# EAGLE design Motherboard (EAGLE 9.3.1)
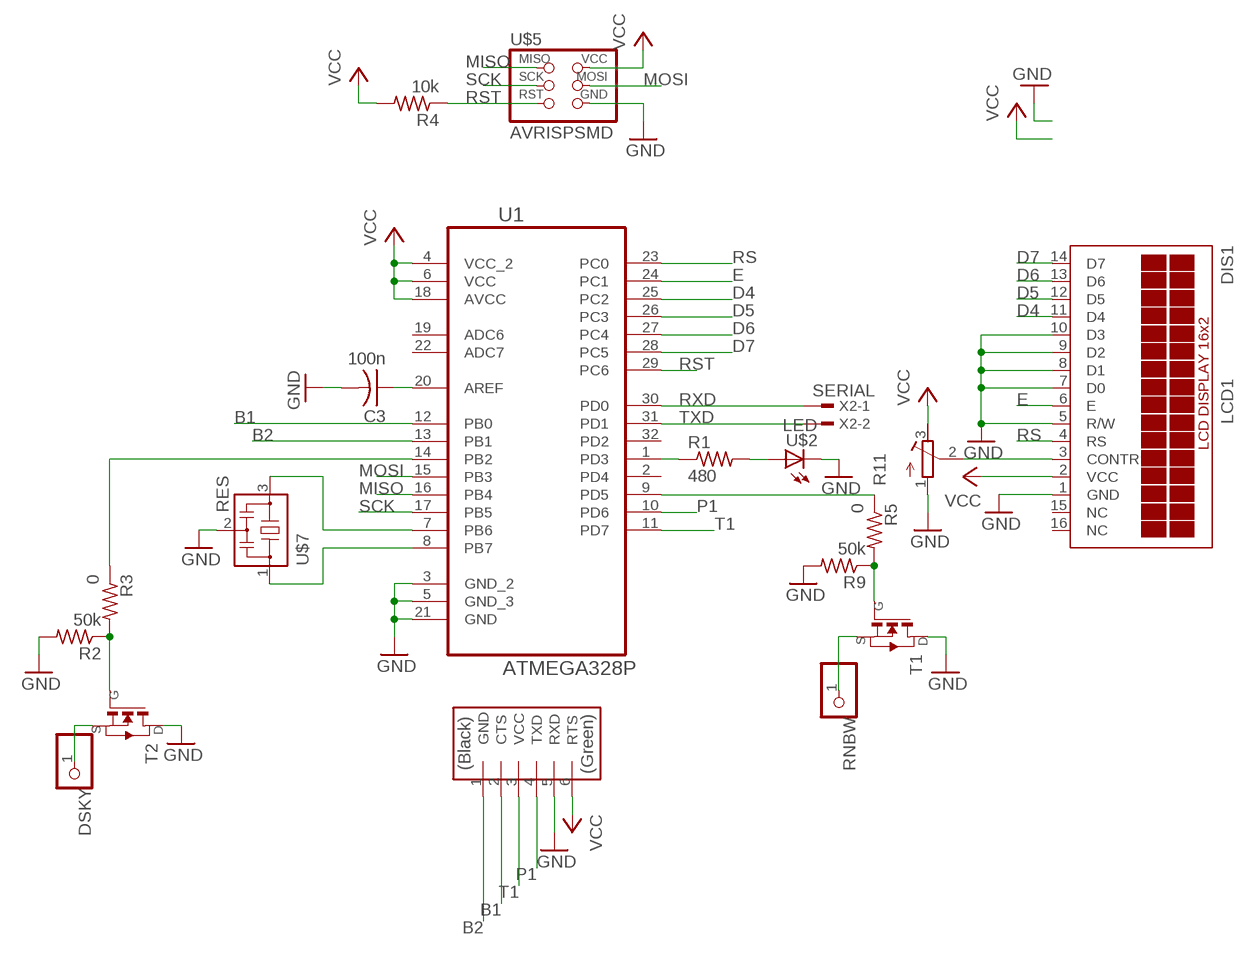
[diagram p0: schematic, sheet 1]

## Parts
C3  100n  CAP-US1206FAB  [C1206FAB]
DIS1  LCD1  TUXGR_16X2_R2  [TUXGR_16X2_R2]
DSKY  PINHD-1X1  [1X01]
R1  480  RES-US1206FAB  [R1206FAB]
R2  50k  RES-US1206FAB  [R1206FAB]
R3  0  RES-US1206FAB  [R1206FAB]
R4  10k  RES-US1206FAB  [R1206FAB]
R5  0  RES-US1206FAB  [R1206FAB]
R9  50k  RES-US1206FAB  [R1206FAB]
R11  R-TRIMM4G/J  [RTRIM4G/J]
RNBW  PINHD-1X1  [1X01]
T1  NMOSFETSOT23  [SOT-23]
T2  NMOSFETSOT23  [SOT-23]
U1  ATMEGA328P  ATMEGA328P-AU  [QFP80P900X900X120-32N]
U$1  FTDI-SMD-HEADER  [1X06SMD]
U$2  LED  LEDFAB1206  [LED1206FAB]
U$5  AVRISPSMD  [2X03SMD]
U$7  RES  RESONATOR  [EFOBM]
X2  SERIAL  TSW-101-07-G-D  [TSW-101-XX-G-D]

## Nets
B1: U1.12(PB0) U$1.2(CTS)
B2: U1.13(PB1) U$1.1(GND)
D4: DIS1.11(D4) U1.25(PC2)
D5: DIS1.12(D5) U1.26(PC3)
D6: DIS1.13(D6) U1.27(PC4)
D7: DIS1.14(D7) U1.28(PC5)
E: DIS1.6(E) U1.24(PC1)
GND: C3.2 DIS1.1(GND) DIS1.5(R/W) DIS1.7(D0) DIS1.8(D1) DIS1.9(D2) DIS1.10(D3) R2.2 R9.2 R11.1(A) T1.1(D) T2.1(D) U1.3(GND_2) U1.5(GND_3) U1.21(GND) U$1.5(RXD) U$2.2(C) U$5.6(GND) U$7.2
MISO: U1.16(PB4) U$5.1(MISO)
MOSI: U1.15(PB3) U$5.4(MOSI)
N$1: DIS1.3(CONTR) R11.2(S)
N$2: U1.7(PB6) U$7.3
N$3: C3.1 U1.20(AREF)
N$4: R1.1 U1.1(PD3)
N$6: R3.1 U1.14(PB2)
N$7: R1.2 U$2.1(A)
N$9: R5.1 U1.9(PD5)
N$11: R2.1 R3.2 T2.3(G)
N$12: R5.2 R9.1 T1.3(G)
N$19: RNBW.1 T1.2(S)
N$21: U1.8(PB7) U$7.1
N$22: DSKY.1 T2.2(S)
P1: U1.10(PD6) U$1.4(TXD)
RS: DIS1.4(RS) U1.23(PC0)
RST: R4.1 U1.29(PC6) U$5.5(RST)
RXD: U1.30(PD0) X2.1
SCK: U1.17(PB5) U$5.3(SCK)
T1: U1.11(PD7) U$1.3(VCC)
TXD: U1.31(PD1) X2.2
VCC: DIS1.2(VCC) R4.2 R11.3(E) U1.4(VCC_2) U1.6(VCC) U1.18(AVCC) U$1.6(RTS) U$5.2(VCC)
Unconnected: DIS1.15(NC) DIS1.16(NC) U1.2(PD4) U1.19(ADC6) U1.22(ADC7) U1.32(PD2)

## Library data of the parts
C3 = fab:CAP-US
DIS1 = lcd16:TUXGR_16X2_R2: Tuxgraphics LCD display 16x2 characters reflective, without background light Source: tuxgr_12x2_r2.pdf; OC_FARNELL: unknown; OC_NEWARK: unknown
DSKY RNBW = pinhead:PINHD-1X1: PIN HEADER
R1-R5 R9 = fab:RES-US: Resistor (US Symbol)
R11 = rcl:R-TRIMM: Trimm resistor; SPICEMODEL: X; SPICEPREFIXL: POT
T1 T2 = fab:NMOSFET: MOS FET
U1 = Atmel_By_element14_Batch_1-00:ATMEGA328P-AU: 8-bit Microcontroller with In-System Programmable Flash; MPN: ATMEGA328P-AU; OC_FARNELL: 1715486; OC_NEWARK: 14R4631; PACKAGE: TQFP-32; SUPPLIER: Atmel
U$1 = fab:FTDI-SMD-HEADER
U$2 = fab:LED: LED
U$5 = fab:AVRISP
U$7 = fab:RESONATOR
X2 = con-samtec:TSW-101-*-G: THROUGH-HOLE .025" SQ POST HEADER; MF: Samtec Inc.; MPN: TSW-101-07-G-D

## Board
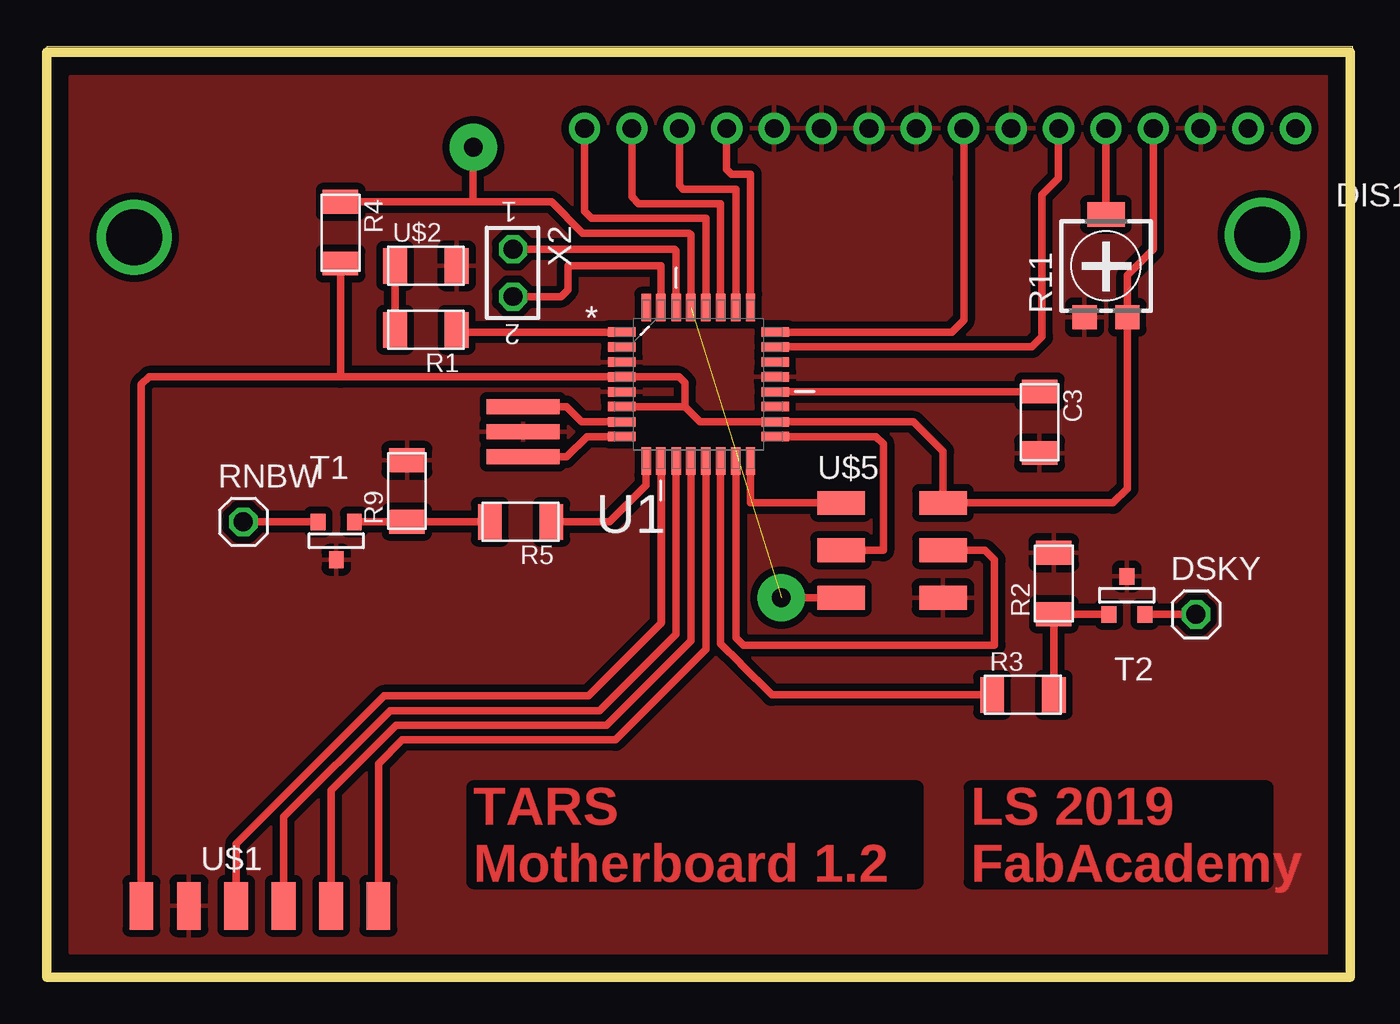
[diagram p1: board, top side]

Size 70 x 49.84 mm. Coordinates in mm from the lower left corner, seen from the top.
Outline: 0,0 70,0 70,49.84 0,49.84 0,0
Copper layers (1*16): Top 0.035mm / dielectric 1.5mm / Bottom 0.035mm
Design rules "default *": minimum track width 16mil, minimum drill 0.35mm, track to track 15mil, track to pad 15mil, pad to pad 15mil, via to via 15mil, smd to smd 15mil, copper to edge 40mil, drill to drill 6mil, minimum pad ring 10mil, minimum via ring 8mil, stop-mask expansion 4mil, vias tented up to drill 0mil, thermal gap 16mil
Milling: 4 lines

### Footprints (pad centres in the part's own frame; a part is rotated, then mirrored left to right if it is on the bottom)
C1206FAB = smd 1.27 x 1.905: 1 -1.651,0; 2 1.651,0
TUXGR_16X2_R2 = drill 1 pad 1.676: 1 -26.92,15.5; 2 -24.38,15.5; 3 -21.84,15.5; 4 -19.3,15.5; 5 -16.76,15.5; 6 -14.22,15.5; 7 -11.68,15.5; 8 -9.14,15.5; 9 -6.6,15.5; 10 -4.06,15.5; 11 -1.52,15.5; 12 1.02,15.5; 13 3.56,15.5; 14 6.1,15.5; 15 -32,15.5; 16 -29.46,15.5
1X01 = drill 1.016 octagon: 1 0,0
R1206FAB = smd 1.27 x 1.905: 1 -1.651,0; 2 1.651,0
RTRIM4G/J = smd 1.3 x 1.3: 1 -1.15,-2.75; 3 1.15,-2.75 | smd 2 x 1.3: 2 0,2.75
SOT-23 = smd 0.787 x 0.889: 1 0.025,-1.016; 2 -0.94,1.016; 3 0.991,1.016
QFP80P900X900X120-32N = smd 1.473 x 0.508: 1 -4.115,2.794; 2 -4.115,2.007; 3 -4.115,1.194; 4 -4.115,0.406; 5 -4.115,-0.406; 6 -4.115,-1.194; 7 -4.115,-2.007; 8 -4.115,-2.794; 17 4.115,-2.794; 18 4.115,-2.007; 19 4.115,-1.194; 20 4.115,-0.406; 21 4.115,0.406; 22 4.115,1.194; 23 4.115,2.007; 24 4.115,2.794 | smd 0.508 x 1.473: 9 -2.794,-4.115; 10 -2.007,-4.115; 11 -1.194,-4.115; 12 -0.406,-4.115; 13 0.406,-4.115; 14 1.194,-4.115; 15 2.007,-4.115; 16 2.794,-4.115; 25 2.794,4.115; 26 2.007,4.115; 27 1.194,4.115; 28 0.406,4.115; 29 -0.406,4.115; 30 -1.194,4.115; 31 -2.007,4.115; 32 -2.794,4.115
1X06SMD = smd 2.54 x 1.27: 1 0,6.35; 2 0,3.81; 3 0,1.27; 4 0,-1.27; 5 0,-3.81; 6 0,-6.35
LED1206FAB = smd 1.27 x 1.905: 1 -1.651,0; 2 1.651,0
2X03SMD = smd 2.54 x 1.27: 1 -2.54,2.54; 2 2.92,2.54; 3 -2.54,0; 4 2.92,0; 5 -2.54,-2.54; 6 2.92,-2.54
EFOBM = smd 0.8 x 3.9: 1 -1.35,0; 2 0,0; 3 1.35,0
TSW-101-XX-G-D = drill 1 pad 1.5 octagon: 1 0.02,-1.27; 2 0.02,1.27

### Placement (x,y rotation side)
C3  53.21,29.72 270 top
DIS1  34.92,60.96 180 top
DSKY  61.59,19.43 0 top
R1  20.32,34.67 180 top
R2  53.98,21.08 90 top
R3  52.32,15.11 0 top
R4  15.75,39.88 270 top
R5  25.4,24.38 180 top
R9  19.3,26.04 90 top
R11  56.77,38.1 0 top
RNBW  10.54,24.38 0 top
T1  15.49,23.37 0 top
T2  57.91,20.45 180 top
U1  34.92,31.75 0 top
U$1  11.43,3.81 270 top
U$2  20.32,38.1 0 top
U$5  45.12,22.86 0 top
U$7  25.53,29.21 90 top
X2  25.02,37.72 180 top

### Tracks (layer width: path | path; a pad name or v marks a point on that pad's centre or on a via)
B1
  Top 0.406: U1.12 34.52,18.01 30,13.49 18.72,13.49 15.24,10 U$1.2
B2
  Top 0.406: U1.13 35.33,17.55 30.48,12.7 19.05,12.7 17.78,11.43 U$1.1
D4
  Top 0.406: DIS1.11 36.45,43.26 36.7,43 37.72,43 U1.25
D5
  Top 0.406: DIS1.12 33.91,42.42 34.11,42.22 36.93,42.22 U1.26
D6
  Top 0.406: U1.27 36.12,41.43 31.73,41.43 31.36,41.79 DIS1.13
D7
  Top 0.406: U1.28 35.33,40.64 29.21,40.64 28.82,41.02 DIS1.14
E
  Top 0.406: DIS1.6 49.15,42.8 49.15,35.17 48.51,34.54 U1.24
GND
  pour Top: 1.27,48.26 68.58,48.26 68.58,1.27 1.27,1.27
H1  (via drill 3)
  other vias: 4.7,39.62
MISO
  Top 0.406: U$5.1 37.72,25.4 U1.16
MOSI
  Top 0.406: U1.15 36.93,18.19 37.34,17.78 50.8,17.78 50.8,22.35 50.29,22.86 U$5.4
N$1
  Top 0.406: R11.2 DIS1.3
N$2
  Top 0.406: U1.7 28.68,29.74 27.86,30.56 U$7.3
N$3
  Top 0.406: C3.1 53.21,31.34 U1.20
N$4
  Top 0.406: U1.1 21.97,34.54 R1.1
N$5  (via drill 1 pad 2.54)
  other vias: 39.37,20.32
N$6
  Top 0.406: U1.14 36.12,17.86 37.15,16.83 37.21,16.76 38.86,15.11 R3.1
N$7
  Top 0.406: R1.2 U$2.1
N$8  (via drill 3)
  other vias: 65.15,39.75
N$9
  Top 0.406: U1.9 32.13,26.34 30.18,24.38 R5.1
N$10  (via drill 1 pad 2.54)
  other vias: 22.86,44.45
N$11
  Top 0.406: T2.3 R2.1 R3.2
N$12
  Top 0.406: T1.3 R9.1 R5.2
N$19
  Top 0.406: T1.2 RNBW.1
N$21
  Top 0.406: U$7.1 27.86,27.86 28.96,28.96 U1.8
N$22
  Top 0.406: T2.2 DSKY.1
P1
  Top 0.406: 32.92,18.95 29.03,15.06 18.07,15.06 10.16,7.15 U$1.4
  Top 0.432: U1.10 32.92,18.95
RS
  Top 0.406: DIS1.4 54.23,42.8 53.34,41.91 53.34,34.29 52.81,33.76 U1.23
RST  (1 unrouted)
  Top 0.406: U1.29 34.52,39.75 34.42,39.85 28.73,39.85 27.05,41.53 22.86,41.53 | R4.1 22.86,41.53 | 22.86,41.53 22.86,44.45 | U$5.5 39.37,20.32
RXD
  Top 0.406: U1.30 33.73,38.91 33.66,38.99 X2.1
SCK
  Top 0.406: U1.17 44.45,28.96 44.83,28.57 44.83,22.86 U$5.3
T1
  Top 0.406: U1.11 33.73,18.36 29.64,14.28 18.4,14.28 12.7,8.58 U$1.3
TXD
  Top 0.406: U1.31 32.92,38.08 arc90 32.89,38.1 27.94,38.1 27.94,36.83 27.56,36.45 X2.2
VCC
  Top 0.406: 34.21,30.56 35.03,29.74 U1.18 46.46,29.74 48.04,28.16 U$5.2 57.15,25.4 57.92,26.17 R11.3 57.92,37.6 59.3,38.98 DIS1.2 | U1.6 34.21,30.56 | 34.21,30.56 34.21,31.83 33.88,32.16 U1.4 15.75,32.16 | 15.75,32.16 5.49,32.16 5.08,31.75 U$1.6 | R4.2 15.75,32.16

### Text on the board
Top: TARS / Motherboard 1.2 | LS 2019 / FabAcademy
